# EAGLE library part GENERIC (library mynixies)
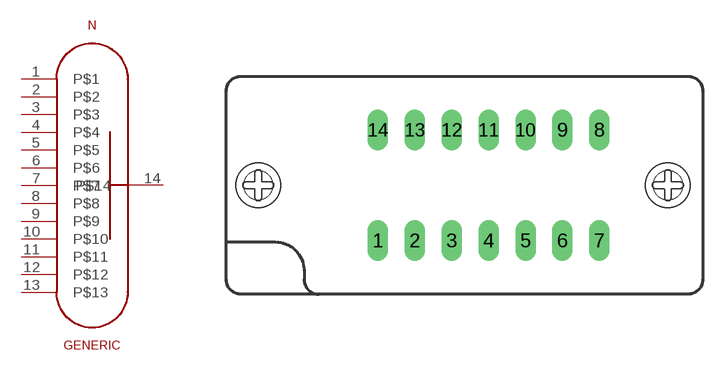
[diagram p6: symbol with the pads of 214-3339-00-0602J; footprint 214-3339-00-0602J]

Designator prefix N

## GENERICZIF  [214-3339-00-0602J]
1  P$1  pas
2  P$2  pas
3  P$3  pas
4  P$4  pas
5  P$5  pas
6  P$6  pas
7  P$7  pas
8  P$8  pas
9  P$9  pas
10  P$10  pas
11  P$11  pas
12  P$12  pas
13  P$13  pas
14  P$14  pas

## Footprint 214-3339-00-0602J (pad centres in mm)
3M TEXTOOL 14 pol. DIP Lever actuated zero insertion force mechanism Hersteller: 3M TEXTOOL Herstellerbez.: 214-3339-00-0602J Farnell Best.-Nr.: 4666290 Source: http://www.3M.com/ehpd
drill 0.9 long: 1 -7.62,-3.81; 2 -5.08,-3.81; 3 -2.54,-3.81; 4 0,-3.81; 5 2.54,-3.81; 6 5.08,-3.81; 7 7.62,-3.81; 8 7.62,3.81; 9 5.08,3.81; 10 2.54,3.81; 11 0,3.81; 12 -2.54,3.81; 13 -5.08,3.81; 14 -7.62,3.81
hole 2 at 12.35,0
hole 2 at -15.85,0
